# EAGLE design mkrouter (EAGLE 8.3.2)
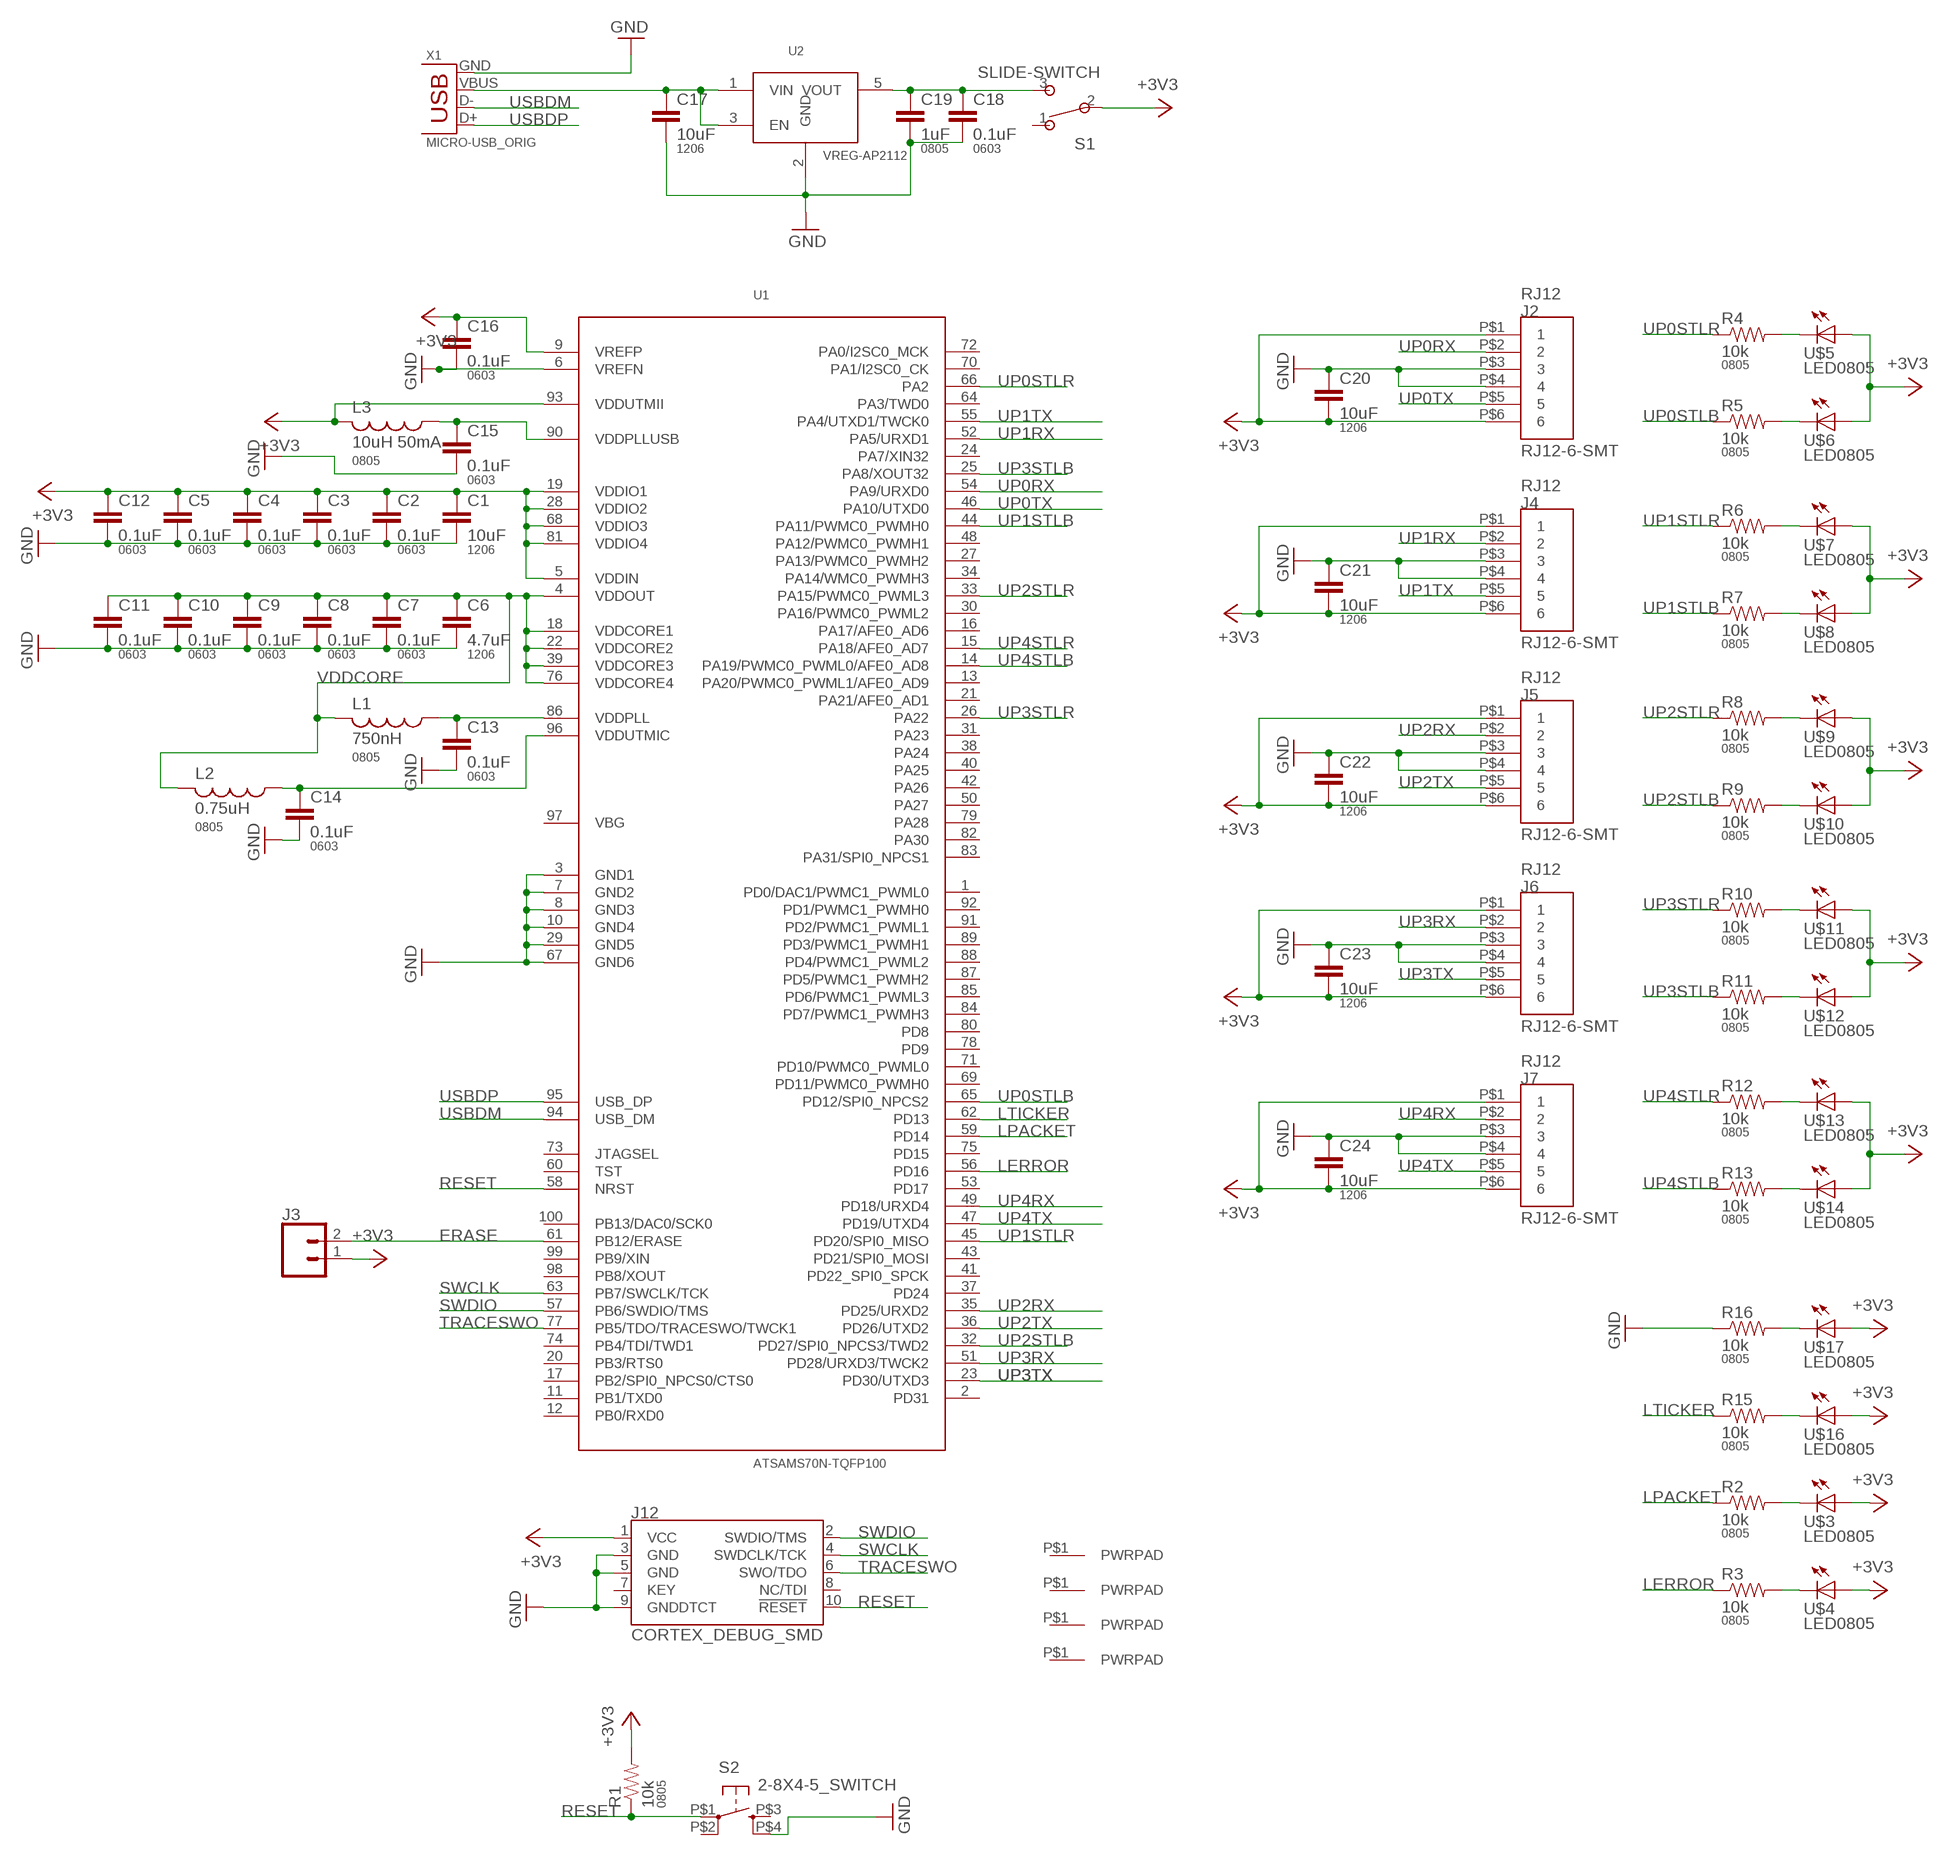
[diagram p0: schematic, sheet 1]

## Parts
C1  10uF  CAP1206  [1206]
C2  0.1uF  CAP0603-CAP  [0603-CAP]
C3  0.1uF  CAP0603-CAP  [0603-CAP]
C4  0.1uF  CAP0603-CAP  [0603-CAP]
C5  0.1uF  CAP0603-CAP  [0603-CAP]
C6  4.7uF  CAP1206  [1206]
C7  0.1uF  CAP0603-CAP  [0603-CAP]
C8  0.1uF  CAP0603-CAP  [0603-CAP]
C9  0.1uF  CAP0603-CAP  [0603-CAP]
C10  0.1uF  CAP0603-CAP  [0603-CAP]
C11  0.1uF  CAP0603-CAP  [0603-CAP]
C12  0.1uF  CAP0603-CAP  [0603-CAP]
C13  0.1uF  CAP0603-CAP  [0603-CAP]
C14  0.1uF  CAP0603-CAP  [0603-CAP]
C15  0.1uF  CAP0603-CAP  [0603-CAP]
C16  0.1uF  CAP0603-CAP  [0603-CAP]
C17  10uF  CAP1206  [1206]
C18  0.1uF  CAP0603-CAP  [0603-CAP]
C19  1uF  CAP0805  [0805]
C20  10uF  CAP1206  [1206]
C21  10uF  CAP1206  [1206]
C22  10uF  CAP1206  [1206]
C23  10uF  CAP1206  [1206]
C24  10uF  CAP1206  [1206]
J2  RJ12-6-SMT  [RJ12-6-SMT]
J3  CONN_021X02_NO_SILK  [1X02_NO_SILK]
J4  RJ12-6-SMT  [RJ12-6-SMT]
J5  RJ12-6-SMT  [RJ12-6-SMT]
J6  RJ12-6-SMT  [RJ12-6-SMT]
J7  RJ12-6-SMT  [RJ12-6-SMT]
J8  PWRPADM3  [PWRPAD_3-25MM]
J9  PWRPADM3  [PWRPAD_3-25MM]
J10  PWRPADM3  [PWRPAD_3-25MM]
J11  PWRPADM3  [PWRPAD_3-25MM]
J12  CORTEX_DEBUG_SMD  [SAMTECH_FTSH-105-01]
L1  750nH  INDUCTOR-0805  [0805]
L2  0.75uH  INDUCTOR-0805  [0805]
L3  10uH 50mA  INDUCTOR-0805  [0805]
R1  10k  RESISTOR0805-RES  [0805]
R2  10k  RESISTOR0805-RES  [0805]
R3  10k  RESISTOR0805-RES  [0805]
R4  10k  RESISTOR0805-RES  [0805]
R5  10k  RESISTOR0805-RES  [0805]
R6  10k  RESISTOR0805-RES  [0805]
R7  10k  RESISTOR0805-RES  [0805]
R8  10k  RESISTOR0805-RES  [0805]
R9  10k  RESISTOR0805-RES  [0805]
R10  10k  RESISTOR0805-RES  [0805]
R11  10k  RESISTOR0805-RES  [0805]
R12  10k  RESISTOR0805-RES  [0805]
R13  10k  RESISTOR0805-RES  [0805]
R15  10k  RESISTOR0805-RES  [0805]
R16  10k  RESISTOR0805-RES  [0805]
S1  SLIDE-SWITCH  [AYZ0102AGRLC]
S2  2-8X4-5_SWITCH  [TACT-SWITCH-KMR6]
U1  ATSAMS70N-TQFP100  [TQFP100-14X14]
U2  VREG-AP2112  [SOT23-5]
U$3  LED0805  [LED0805]
U$4  LED0805  [LED0805]
U$5  LED0805  [LED0805]
U$6  LED0805  [LED0805]
U$7  LED0805  [LED0805]
U$8  LED0805  [LED0805]
U$9  LED0805  [LED0805]
U$10  LED0805  [LED0805]
U$11  LED0805  [LED0805]
U$12  LED0805  [LED0805]
U$13  LED0805  [LED0805]
U$14  LED0805  [LED0805]
U$16  LED0805  [LED0805]
U$17  LED0805  [LED0805]
X1  MICRO-USB_ORIG  [DX4R005HJ5]

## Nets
+3V3: C1.1 C2.1 C3.1 C4.1 C5.1 C12.1 C16.1 C20.2 C21.2 C22.2 C23.2 C24.2 J2.P$1 J2.P$6 J3.1 J4.P$1 J4.P$6 J5.P$1 J5.P$6 J6.P$1 J6.P$6 J7.P$1 J7.P$6 J12.1(VCC) L3.2 R1.2 S1.2 U1.5(VDDIN) U1.9(VREFP) U1.19(VDDIO1) U1.28(VDDIO2) U1.68(VDDIO3) U1.81(VDDIO4) U1.93(VDDUTMII) U$3.1(A) U$4.1(A) U$5.1(A) U$6.1(A) U$7.1(A) U$8.1(A) U$9.1(A) U$10.1(A) U$11.1(A) U$12.1(A) U$13.1(A) U$14.1(A) U$16.1(A) U$17.1(A)
ERASE: J3.2 U1.61(PB12/ERASE)
GND: C1.2 C2.2 C3.2 C4.2 C5.2 C6.2 C7.2 C8.2 C9.2 C10.2 C11.2 C12.2 C13.2 C14.2 C15.2 C16.2 C17.2 C18.2 C19.2 C20.1 C21.1 C22.1 C23.1 C24.1 J2.P$3 J2.P$4 J4.P$3 J4.P$4 J5.P$3 J5.P$4 J6.P$3 J6.P$4 J7.P$3 J7.P$4 J12.3(GND) J12.5(GND) J12.9(GNDDTCT) R16.1 S2.P$4(S1) U1.3(GND1) U1.6(VREFN) U1.7(GND2) U1.8(GND3) U1.10(GND4) U1.29(GND5) U1.67(GND6) U2.2(GND) X1.GND
LERROR: R3.1 U1.56(PD16)
LPACKET: R2.1 U1.59(PD14)
LTICKER: R15.1 U1.62(PD13)
N$1: C13.1 L1.1 U1.86(VDDPLL)
N$2: R7.2 U$8.2(C)
N$3: C14.1 L2.1 U1.96(VDDUTMIC)
N$4: C17.1 U2.1(VIN) U2.3(EN) X1.VBUS
N$5: C15.1 L3.1 U1.90(VDDPLLUSB)
N$6: R5.2 U$6.2(C)
N$7: C18.1 C19.1 S1.3 U2.5(VOUT)
N$8: R4.2 U$5.2(C)
N$9: R6.2 U$7.2(C)
N$10: R9.2 U$10.2(C)
N$11: R8.2 U$9.2(C)
N$12: R11.2 U$12.2(C)
N$13: R10.2 U$11.2(C)
N$14: R13.2 U$14.2(C)
N$15: R12.2 U$13.2(C)
N$16: R2.2 U$3.2(C)
N$17: R3.2 U$4.2(C)
N$22: R15.2 U$16.2(C)
N$23: R16.2 U$17.2(C)
RESET: J12.10(!RESET) R1.1 S2.P$1(P) U1.58(NRST)
SWCLK: J12.4(SWDCLK/TCK) U1.63(PB7/SWCLK/TCK)
SWDIO: J12.2(SWDIO/TMS) U1.57(PB6/SWDIO/TMS)
TRACESWO: J12.6(SWO/TDO) U1.77(PB5/TDO/TRACESWO/TWCK1)
UP0RX: J2.P$2 U1.54(PA9/URXD0)
UP0STLB: R5.1 U1.65(PD12/SPI0_NPCS2)
UP0STLR: R4.1 U1.66(PA2)
UP0TX: J2.P$5 U1.46(PA10/UTXD0)
UP1RX: J4.P$2 U1.52(PA5/URXD1)
UP1STLB: R7.1 U1.44(PA11/PWMC0_PWMH0)
UP1STLR: R6.1 U1.45(PD20/SPI0_MISO)
UP1TX: J4.P$5 U1.55(PA4/UTXD1/TWCK0)
UP2RX: J5.P$2 U1.35(PD25/URXD2)
UP2STLB: R9.1 U1.32(PD27/SPI0_NPCS3/TWD2)
UP2STLR: R8.1 U1.33(PA15/PWMC0_PWML3)
UP2TX: J5.P$5 U1.36(PD26/UTXD2)
UP3RX: J6.P$2 U1.51(PD28/URXD3/TWCK2)
UP3STLB: R11.1 U1.25(PA8/XOUT32)
UP3STLR: R10.1 U1.26(PA22)
UP3TX: J6.P$5 U1.23(PD30/UTXD3)
UP4RX: J7.P$2 U1.49(PD18/URXD4)
UP4STLB: R13.1 U1.14(PA19/PWMC0_PWML0/AFE0_AD8)
UP4STLR: R12.1 U1.15(PA18/AFE0_AD7)
UP4TX: J7.P$5 U1.47(PD19/UTXD4)
USBDM: U1.94(USB_DM) X1.D-
USBDP: U1.95(USB_DP) X1.D+
VDDCORE: C6.1 C7.1 C8.1 C9.1 C10.1 C11.1 L1.2 L2.2 U1.4(VDDOUT) U1.18(VDDCORE1) U1.22(VDDCORE2) U1.39(VDDCORE3) U1.76(VDDCORE4)
Unconnected: J8.P$1(PWRPAD) J9.P$1(PWRPAD) J10.P$1(PWRPAD) J11.P$1(PWRPAD) J12.7(KEY) J12.8(NC/TDI) S1.1 S2.P$2(P1) S2.P$3(S) U1.1(PD0/DAC1/PWMC1_PWML0) U1.2(PD31) U1.11(PB1/TXD0) U1.12(PB0/RXD0) U1.13(PA20/PWMC0_PWML1/AFE0_AD9) U1.16(PA17/AFE0_AD6) U1.17(PB2/SPI0_NPCS0/CTS0) U1.20(PB3/RTS0) U1.21(PA21/AFE0_AD1) U1.24(PA7/XIN32) U1.27(PA13/PWMC0_PWMH2) U1.30(PA16/PWMC0_PWML2) U1.31(PA23) U1.34(PA14/WMC0_PWMH3) U1.37(PD24) U1.38(PA24) U1.40(PA25) U1.41(PD22_SPI0_SPCK) U1.42(PA26) U1.43(PD21/SPI0_MOSI) U1.48(PA12/PWMC0_PWMH1) U1.50(PA27) U1.53(PD17) U1.60(TST) U1.64(PA3/TWD0) U1.69(PD11/PWMC0_PWMH0) U1.70(PA1/I2SC0_CK) U1.71(PD10/PWMC0_PWML0) U1.72(PA0/I2SC0_MCK) U1.73(JTAGSEL) U1.74(PB4/TDI/TWD1) U1.75(PD15) U1.78(PD9) U1.79(PA28) U1.80(PD8) U1.82(PA30) U1.83(PA31/SPI0_NPCS1) U1.84(PD7/PWMC1_PWMH3) U1.85(PD6/PWMC1_PWML3) U1.87(PD5/PWMC1_PWMH2) U1.88(PD4/PWMC1_PWML2) U1.89(PD3/PWMC1_PWMH1) U1.91(PD2/PWMC1_PWML1) U1.92(PD1/PWMC1_PWMH0) U1.97(VBG) U1.98(PB8/XOUT) U1.99(PB9/XIN) U1.100(PB13/DAC0/SCK0)

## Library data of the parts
C1 C6 C17 C20-C24 = borkedlabs-passives:CAP: Capacitor; PACKAGE: 1206
C2-C5 C7-C16 C18 = borkedlabs-passives:CAP: Capacitor; PACKAGE: 0603
C19 = borkedlabs-passives:CAP: Capacitor; PACKAGE: 0805
J2 J4-J7 = connector:RJ12-6-SMT
J3 = SparkFun-Connectors:CONN_02: Multi connection point. Often used as Generic Header-pin footprint for 0.1 inch spaced/style header connections
J8-J11 = power:PWRPAD
J12 = SparkFun-Connectors:CORTEX_DEBUG: Cortex Debug Connector - 10 pin Supports JTAG debug, Serial Wire debug, and Serial Wire Viewer. PTH and SMD connector options available. General Connector Information Products: PTH Connector -via Digi-Key SparkFun PSoc SparkFun T
L1-L3 = borkedlabs-passives:INDUCTOR; PACKAGE: 0805
R1-R13 R15 R16 = borkedlabs-passives:RESISTOR: Resistor; PACKAGE: 0805
S1 = fab:SLIDE-SWITCH: SMD slide-switch AYZ0102AGRLC as found in the fablab inventory. Includes the mounting holes. Made by Zaerc.
S2 = fab:2-8X4-5_SWITCH
U1 = atsam:ATSAMS70N-TQFP100
U2 = power:VREG-AP2112
U$3-U$14 U$16 U$17 = lights:LED: LED
X1 = fab:MICRO-USB: SMD micro USB connector as found in the fablab inventory. Three footprint variants included: original, as described by manufacturer's datasheet for milling with the 1/100" bit for milling with the 1/64" bit Made by Zaerc.

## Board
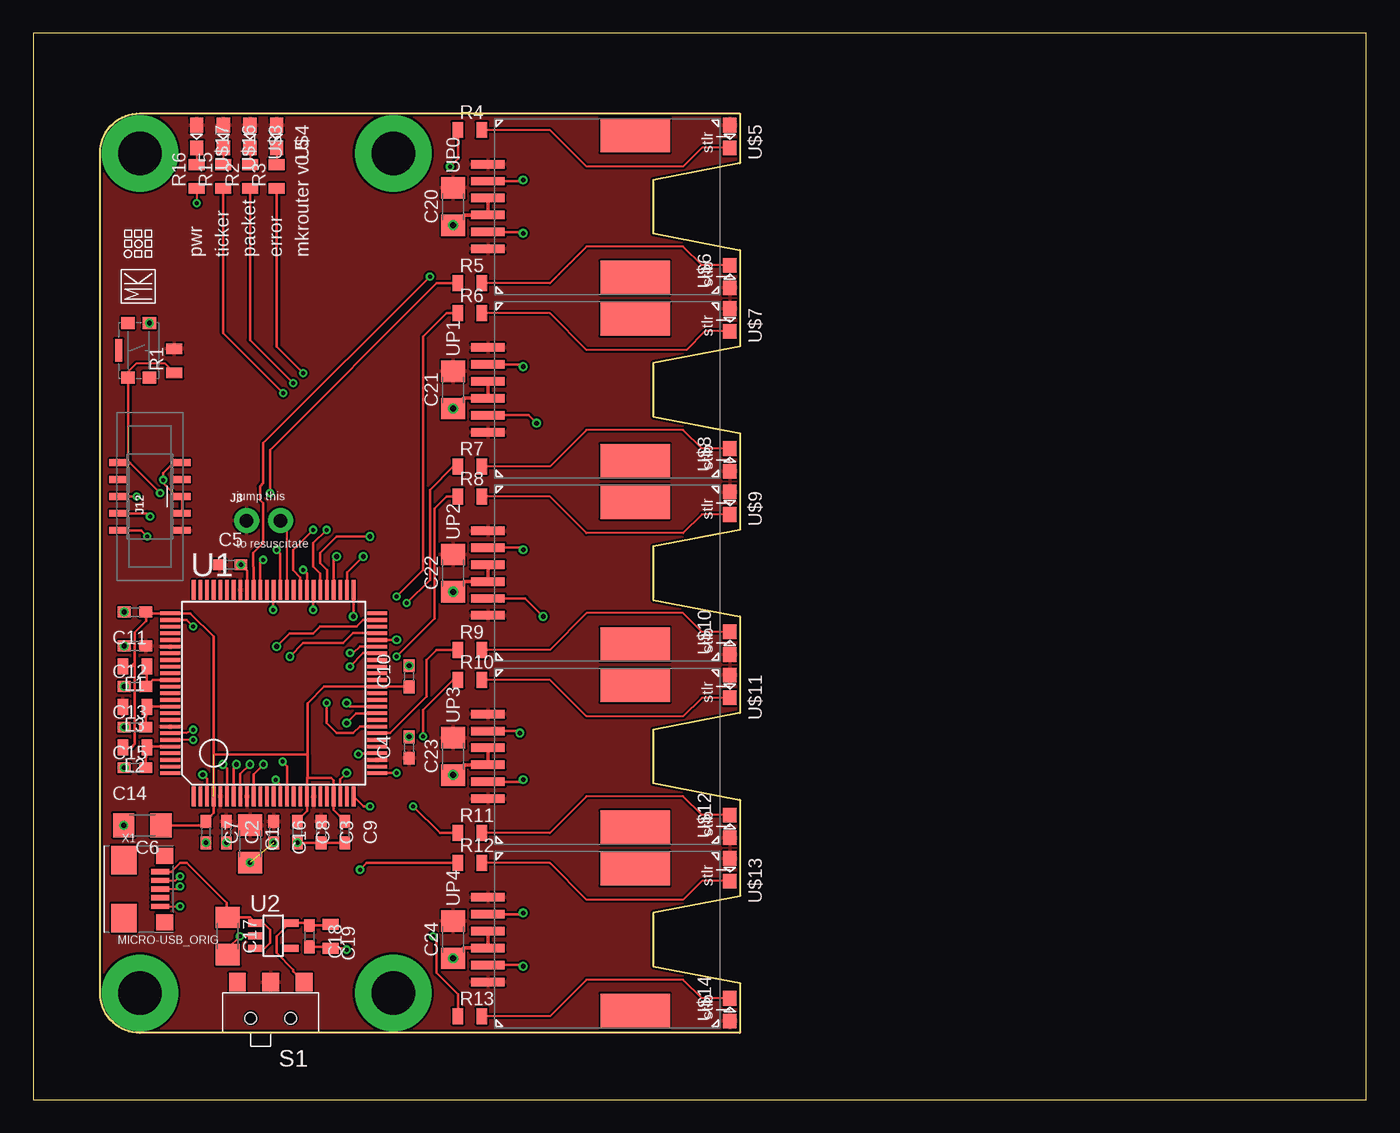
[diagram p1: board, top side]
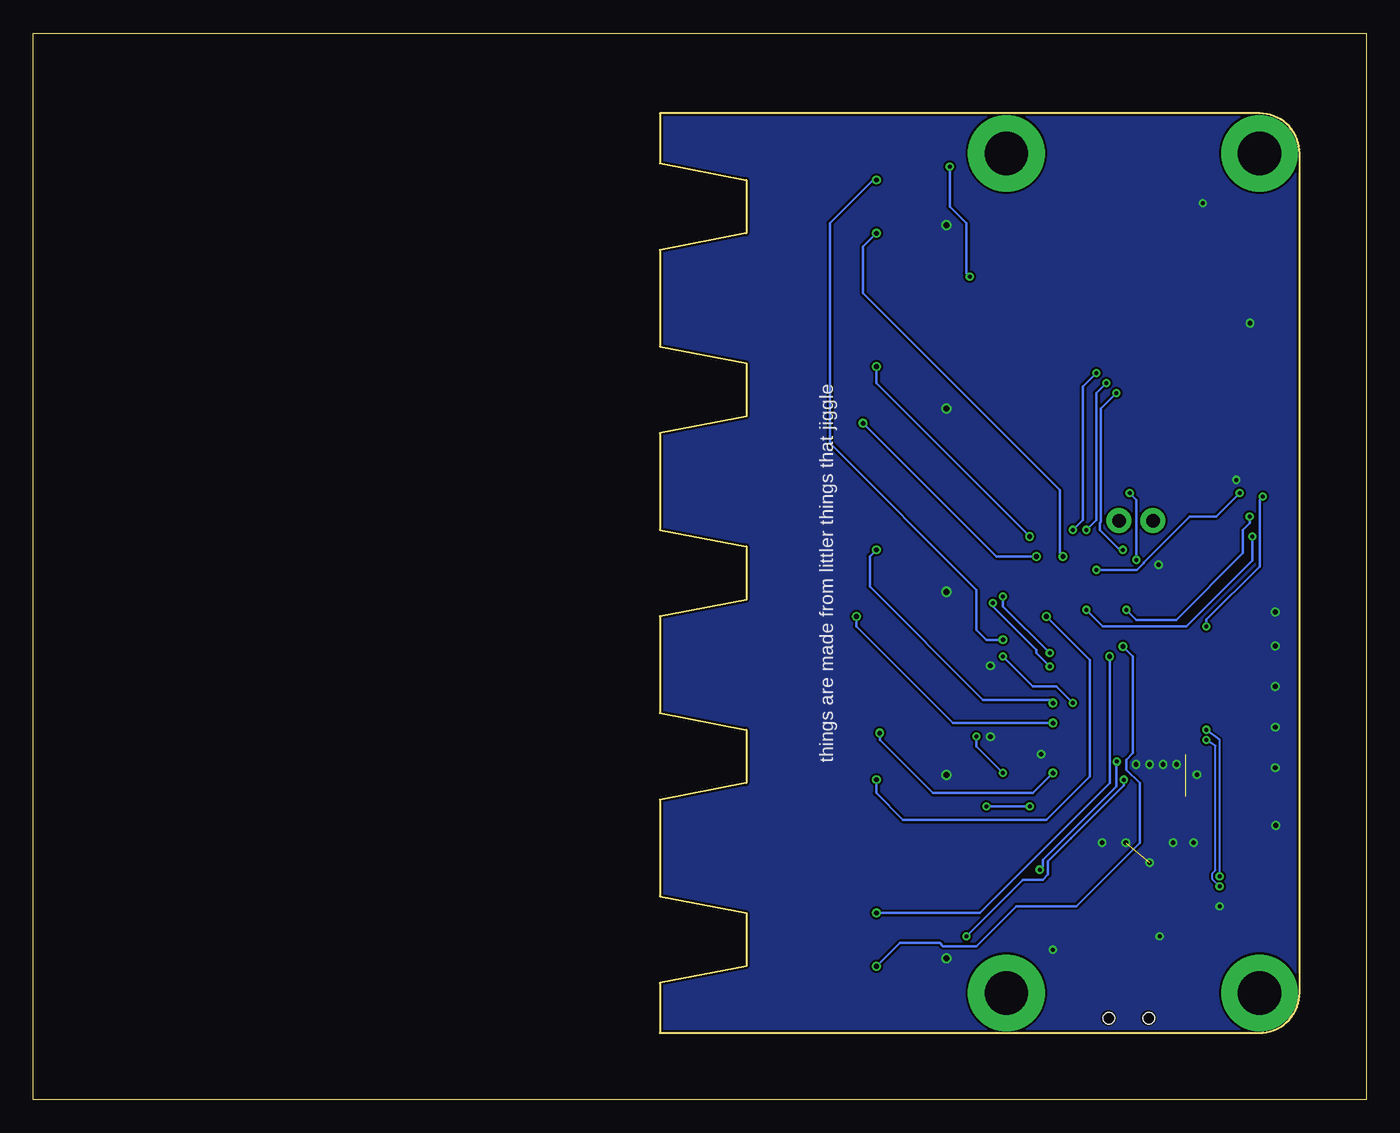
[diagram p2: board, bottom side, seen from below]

Size 100 x 80 mm. Coordinates in mm from the lower left corner, seen from the top.
Outline: 0,0 100,0 100,80 0,80 0,0
Outline: 8,74 53,74 53,70.25 46.5,69 46.5,65 53,63.75 53,56.5 46.5,55.25 46.5,51.25 53,50 53,42.75 46.5,41.5 46.5,37.5 53,36.25 53,29 46.5,27.75 46.5,23.75 53,22.5 53,15.25 46.5,14 46.5,10 53,8.75 53,5 8,5 arc-90 5,8 5,71 arc-90 8,74
Copper layers (1*16): Top 0.035mm / dielectric 1.5mm / Bottom 0.035mm
Design rules "default *": minimum track width 6mil, minimum drill 0.3mm, track to track 6mil, track to pad 6mil, pad to pad 6mil, via to via 6mil, smd to smd 6mil, copper to edge 6mil, drill to drill 6mil, minimum pad ring 10mil, minimum via ring 6mil, stop-mask expansion 4mil, vias tented up to drill 20mil, thermal gap 6mil

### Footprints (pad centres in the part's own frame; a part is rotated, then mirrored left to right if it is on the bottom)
1206 = smd 1.6 x 1.8: 1 -1.4,0; 2 1.4,0
0603-CAP = smd 0.96 x 0.8: 1 -0.8,0; 2 0.8,0
0805 = smd 0.8 x 1.2: 1 -0.9,0; 2 0.9,0
RJ12-6-SMT = smd 0.635 x 2.54: P$1 -3.175,17.399; P$2 -1.905,17.399; P$3 -0.635,17.399; P$4 0.635,17.399; P$5 1.905,17.399; P$6 3.175,17.399 | smd 2.54 x 5.207: P$7 -5.334,6.35; P$8 5.334,6.35
1X02_NO_SILK = drill 1.016 pad 1.88: 1 0,0; 2 2.54,0
PWRPAD_3-25MM = drill 3.25 pad 5.75: P$1 0,0
SAMTECH_FTSH-105-01 = smd 0.508 x 1.27: 1 -2.54,-2.413; 2 -2.54,2.413; 3 -1.27,-2.413; 4 -1.27,2.413; 5 0,-2.413; 6 0,2.413; 7 1.27,-2.413; 8 1.27,2.413; 9 2.54,-2.413; 10 2.54,2.413
AYZ0102AGRLC = smd 1.27 x 1.397: 1 2.5,-2.3; 2 0,-2.3; 3 -2.5,-2.3 | hole 0.85: -1.5,0.4; 1.5,0.4
TACT-SWITCH-KMR6 = smd 0.9 x 1: P$1 -2.05,0.8; P$2 2.05,0.8; P$3 -2.05,-0.8; P$4 2.05,-0.8 | smd 1.7 x 0.55: P$5 0,1.5
TQFP100-14X14 = smd 0.27 x 1.5: 1 -6,-7.75; 2 -5.5,-7.75; 3 -5,-7.75; 4 -4.5,-7.75; 5 -4,-7.75; 6 -3.5,-7.75; 7 -3,-7.75; 8 -2.5,-7.75; 9 -2,-7.75; 10 -1.5,-7.75; 11 -1,-7.75; 12 -0.5,-7.75; 13 0,-7.75; 14 0.5,-7.75; 15 1,-7.75; 16 1.5,-7.75; 17 2,-7.75; 18 2.5,-7.75; 19 3,-7.75; 20 3.5,-7.75; 21 4,-7.75; 22 4.5,-7.75; 23 5,-7.75; 24 5.5,-7.75; 25 6,-7.75; 51 6,7.75; 52 5.5,7.75; 53 5,7.75; 54 4.5,7.75; 55 4,7.75; 56 3.5,7.75; 57 3,7.75; 58 2.5,7.75; 59 2,7.75; 60 1.5,7.75; 61 1,7.75; 62 0.5,7.75; 63 0,7.75; 64 -0.5,7.75; 65 -1,7.75; 66 -1.5,7.75; 67 -2,7.75; 68 -2.5,7.75; 69 -3,7.75; 70 -3.5,7.75; 71 -4,7.75; 72 -4.5,7.75; 73 -5,7.75; 74 -5.5,7.75; 75 -6,7.75 | smd 1.5 x 0.27: 26 7.75,-6; 27 7.75,-5.5; 28 7.75,-5; 29 7.75,-4.5; 30 7.75,-4; 31 7.75,-3.5; 32 7.75,-3; 33 7.75,-2.5; 34 7.75,-2; 35 7.75,-1.5; 36 7.75,-1; 37 7.75,-0.5; 38 7.75,0; 39 7.75,0.5; 40 7.75,1; 41 7.75,1.5; 42 7.75,2; 43 7.75,2.5; 44 7.75,3; 45 7.75,3.5; 46 7.75,4; 47 7.75,4.5; 48 7.75,5; 49 7.75,5.5; 50 7.75,6; 76 -7.75,6; 77 -7.75,5.5; 78 -7.75,5; 79 -7.75,4.5; 80 -7.75,4; 81 -7.75,3.5; 82 -7.75,3; 83 -7.75,2.5; 84 -7.75,2; 85 -7.75,1.5; 86 -7.75,1; 87 -7.75,0.5; 88 -7.75,0; 89 -7.75,-0.5; 90 -7.75,-1; 91 -7.75,-1.5; 92 -7.75,-2; 93 -7.75,-2.5; 94 -7.75,-3; 95 -7.75,-3.5; 96 -7.75,-4; 97 -7.75,-4.5; 98 -7.75,-5; 99 -7.75,-5.5; 100 -7.75,-6
SOT23-5 = smd 0.533 x 1.194: 1 -0.95,-1.306; 2 0,-1.306; 3 0.95,-1.306; 4 0.95,1.306; 5 -0.95,1.306
LED0805 = smd 1.1 x 1: 1 -0.85,0; 2 0.85,0
DX4R005HJ5 = smd 0.4 x 1.35: D+ 0,1.6; D- -0.65,1.6; GND 1.3,1.6; ID 0.65,1.6; VBUS -1.3,1.6 | smd 1.2 x 1.3: GND@1 -2.5,1.95; GND@2 2.5,1.95 | smd 2.15 x 1.9: GND@3 -2.175,-1.1; GND@4 2.175,-1.1

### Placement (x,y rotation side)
C1  16.26,19.18 270 top
C2  14.48,20.07 270 top
C3  21.59,20.07 270 top
C4  28.19,26.42 90 top
C5  14.77,40.12 0 top
C6  8.18,20.57 180 top
C7  12.95,20.07 270 top
C8  19.81,20.07 270 top
C9  23.37,20.07 270 top
C10  28.19,31.75 90 top
C11  7.62,36.58 180 top
C12  7.62,34.04 180 top
C13  7.62,30.99 180 top
C14  7.62,24.89 180 top
C15  7.62,27.94 180 top
C16  18.03,20.07 270 top
C17  14.58,12.26 270 top
C18  20.72,12.26 270 top
C19  22.29,12.25 270 top
C20  31.5,67 90 top
C21  31.5,53.25 90 top
C22  31.5,39.5 90 top
C23  31.5,25.75 90 top
C24  31.5,12 90 top
J2  51.5,67 90 top
J3  16,43.43 0 top
J4  51.5,53.25 90 top
J5  51.5,39.5 90 top
J6  51.5,25.75 90 top
J7  51.5,12 90 top
J8  8,8 0 top
J9  27,8 0 top
J10  27,71 0 top
J11  8,71 0 top
J12  8.75,45.25 90 top
L1  7.62,32.51 180 top
L2  7.62,26.42 180 top
L3  7.62,29.46 180 top
R1  10.58,55.43 90 top
R2  16.25,69.25 90 top
R3  18.25,69.25 90 top
R4  32.75,72.75 0 top
R5  32.75,61.25 0 top
R6  32.75,59 0 top
R7  32.75,47.5 0 top
R8  32.75,45.25 0 top
R9  32.75,33.75 0 top
R10  32.75,31.5 0 top
R11  32.75,20 0 top
R12  32.75,17.75 0 top
R13  32.75,6.25 0 top
R15  14.25,69.25 90 top
R16  12.25,69.25 90 top
S1  17.81,6.5 180 top
S2  7.9,56.21 90 top
U1  18.03,30.48 0 top
U2  18.01,12.29 270 top
U$1  [CBA-SILK-LOGO]  7.87,64.22 90 top
U$2  [MK-LOGO-SILK]  7.87,61.01 90 top
U$3  16.25,72.25 270 top
U$4  18.25,72.25 270 top
U$5  52.25,72.25 270 top
U$6  52.25,61.75 90 top
U$7  52.25,58.5 270 top
U$8  52.25,48 90 top
U$9  52.25,44.75 270 top
U$10  52.25,34.25 90 top
U$11  52.25,31 270 top
U$12  52.25,20.5 90 top
U$13  52.25,17.25 270 top
U$14  52.25,6.75 90 top
U$16  14.25,72.25 270 top
U$17  12.25,72.25 270 top
X1  7.9,15.8 270 top

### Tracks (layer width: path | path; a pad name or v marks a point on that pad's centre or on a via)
+3V3
  pour Top (rank 2): 5,74 5,5 53,5 53,74
ERASE
  Top 0.152: U1.61 19.03,42.94 J3.2
GND  (via drill 0.3, 0.35, 0.45)  (1 unrouted)
  Top 0.152: X1.GND v11,14.5 | R16.1 v12.25,67.25
  Top 0.2: U2.2 15.54,12.29 v15.5,12.25
  Top 0.203: U1.3 13.03,24.05 v12.7,24.38 | U1.6 14.53,24.84 v14.22,25.15 | U1.7 15.03,24.94 v15.24,25.15 | U1.8 15.53,24.42 v16.26,25.15 | U1.10 16.53,24.41 v17.27,25.15 | U1.29 24.46,25.98 v24.38,25.91 | C9.2 C3.2 C8.2 | C17.2 14.58,11.33 v15.5,12.25 | C18.2 22.18,11.46 C19.2 23.4,11.35 v23.5,11.25 | J12.3 J12.5 10.75,45.25 9.75,46.25 v9.75,46.5 9.75,47 10.54,47.79 J12.9 | U1.67 16.03,39.66 C5.2
  Top 0.254: J2.P$4 J2.P$3 32.27,66.36 C20.1 | J4.P$4 J4.P$3 32.27,52.62 C21.1 | J5.P$4 J5.P$3 32.27,38.87 C22.1 | J6.P$4 J6.P$3 32.27,25.11 C23.1 | J7.P$4 J7.P$3 32.27,11.37 C24.1
  other vias: 6.82,36.58 6.82,34.04 6.82,30.99 6.82,27.94 6.82,24.89 15.57,40.12 6.78,20.57 12.95,19.27 14.48,19.27 16.26,17.78 18.03,19.27 19.81,19.27 28.19,27.22 28.19,32.55 8.7,58.26 31.5,65.6 31.5,51.85 31.5,38.1 31.5,24.35 31.5,10.6
  pour Bottom: 5,74 53,74 53,5 5,5
LERROR  (via drill 0.3)
  Top 0.203: R3.1 18.25,56.5 v20.25,54.5 | v22,42.75 21,41.75 21,40 21.53,39.47 U1.56
  Bottom 0.203: v20.25,54.5 21.25,53.5 21.25,43.5 v22,42.75
LPACKET  (via drill 0.3)
  Top 0.203: R2.1 16.25,57 v19.5,53.75 | v21,42.75 19.5,41.25 19.5,39.71 20.03,39.18 U1.59
  Bottom 0.203: v19.5,53.75 20.25,53 20.25,43.5 v21,42.75
LTICKER  (via drill 0.3)
  Top 0.203: U1.62 18.53,40.97 v18.25,41.25 | v18.75,53 14.25,57.5 R15.1
  Bottom 0.203: v18.25,41.25 18.5,41.25 20,42.75 20,43.25 19.89,43.35 19.89,51.86 v18.75,53
N$1
  Top 0.203: 8.52,31.04 L1.1 | 8.52,31.04 C13.1 | U1.86 8.96,31.48 8.52,31.04
N$2
  Top 0.152: U$8.2 50.15,48.85 48.75,50.25 41.5,50.25 38.75,47.5 R7.2
N$3
  Top 0.203: U1.96 8.58,26.48 L2.1 8.47,26.37 C14.1
N$4
  Top 0.2: X1.VBUS 10.35,17.1 11,17.75 11.5,17.75 14.5,14.75 14.5,13.75 C17.1 16.28,13.66 U2.1 17.26,13.24 17.75,12.75 17.75,11.75 17.25,11.25 16.79,11.25 U2.3
N$5
  Top 0.203: U1.90 8.54,29.48 L3.1 8.47,29.41 C15.1
N$6
  Top 0.152: U$6.2 50.15,62.6 48.75,64 41.5,64 38.75,61.25 R5.2
N$7
  Top 0.2: C19.1 22.2,13.06 C18.1 20.54,13.24 U2.5 19.24,13.24 18.25,12.25 18.25,11 19.5,9.75 19.5,9.61 S1.3
N$8
  Top 0.152: U$5.2 50.15,71.4 48.75,70 41.5,70 38.75,72.75 R4.2
N$9
  Top 0.152: U$7.2 50.4,57.65 49,56.25 41.5,56.25 38.75,59 R6.2
N$10
  Top 0.152: U$10.2 50.15,35.1 48.75,36.5 41.5,36.5 38.75,33.75 R9.2
N$11
  Top 0.152: U$9.2 50.15,43.9 48.75,42.5 41.5,42.5 38.75,45.25 R8.2
N$12
  Top 0.152: U$12.2 50.15,21.35 48.75,22.75 41.5,22.75 38.75,20 R11.2
N$13
  Top 0.152: U$11.2 50.15,30.15 48.75,28.75 41.5,28.75 38.75,31.5 R10.2
N$14
  Top 0.152: U$14.2 50.15,7.6 48.75,9 41.5,9 38.75,6.25 R13.2
N$15
  Top 0.152: U$13.2 50.15,16.4 48.75,15 41.5,15 38.75,17.75 R12.2
N$16
  Top 0.152: U$3.2 R2.2
N$17
  Top 0.152: U$4.2 R3.2
N$22
  Top 0.152: U$16.2 R15.2
N$23
  Top 0.152: U$17.2 R16.2
RESET  (via drill 0.3)
  Top 0.152: S2.P$1 7.1,54.6 7.75,55.25 9.86,55.25 R1.1
  Top 0.203: U1.58 20.53,39.47 v20.25,39.75 | 7.25,47.75 v9.5,45.5 | 7.25,47.75 6.38,47.75 J12.10 | S2.P$1 7.1,47.9 7.25,47.75
  Bottom 0.203: v20.25,39.75 17.21,39.75 16.69,40.27 16.69,40.31 13.25,43.75 11.25,43.75 v9.5,45.5
SWCLK  (via drill 0.3)
  Top 0.203: J12.4 8.52,43.98 v8.75,43.75 | v18,36.75 18,38.2 U1.63
  Bottom 0.203: v8.75,43.75 8.75,43.25 9.25,42.75 9.25,41 14.25,36 17.25,36 v18,36.75
SWDIO  (via drill 0.3)
  Top 0.203: J12.2 8.1,42.71 v8.56,42.25 | v21,36.75 21,38.2 U1.57
  Bottom 0.203: v8.56,42.25 8.56,40.44 13.5,35.5 19.75,35.5 v21,36.75
TRACESWO  (via drill 0.3)
  Top 0.203: U1.77 11.49,35.98 v11.99,35.49 | v7.75,45.25 J12.6
  Bottom 0.203: v11.99,35.49 11.99,36.01 8,40 8,45 v7.75,45.25
UP0RX  (via drill 0.35)
  Top 0.203: J2.P$2 36.66,65.09 v36.75,65 | U1.54 22.53,40.53 v22.75,40.75
  Bottom 0.203: v36.75,65 37.75,64 37.75,60.5 23,45.75 23,41 v22.75,40.75
UP0STLB  (via drill 0.3)
  Top 0.203: U1.65 17.03,40.28 v17.25,40.5 | v17.75,45.5 17.75,48.75 30.25,61.25 R5.1
  Bottom 0.203: v17.25,40.5 17.25,45 v17.75,45.5
UP0STLR  (via drill 0.3)
  Top 0.203: R4.1 31.85,70.6 v31.25,70 | v29.75,61.75 17.25,49.25 17.25,46.25 17,46 17,45 17.25,44.75 17.25,41.75 16.5,41 16.5,40 16.53,39.97 U1.66
  Bottom 0.203: v31.25,70 31.25,67 30,65.75 30,62 v29.75,61.75
UP0TX  (via drill 0.35)
  Top 0.203: J2.P$5 36.66,68.91 v36.75,69 | v27.25,34.5 25.8,34.5 U1.46
  Bottom 0.203: v36.75,69 37,69 40.25,65.75 40.25,49.25 29.25,38.25 29.25,35.25 28.5,34.5 v27.25,34.5
UP1RX  (via drill 0.35)
  Top 0.203: J4.P$2 37.16,51.34 v37.75,50.75 | U1.52 23.53,39.53 v24.75,40.75
  Bottom 0.203: v37.75,50.75 27.75,40.75 v24.75,40.75
UP1STLB  (via drill 0.3)
  Top 0.203: R7.1 31.5,47.5 29.75,45.75 29.75,39 v28,37.25 | v23.75,32.5 24.75,33.5 25.76,33.5 U1.44
  Bottom 0.203: v28,37.25 28,37 24.75,33.75 24.75,33.5 v23.75,32.5
UP1STLR  (via drill 0.3)
  Top 0.203: R6.1 31,59 29.25,57.25 29.25,39.75 v27.25,37.75 | v23.75,33.5 24,33.5 24.5,34 25.76,34 U1.45
  Bottom 0.203: v27.25,37.75 27.25,37 v23.75,33.5
UP1TX  (via drill 0.35)
  Top 0.203: J4.P$5 36.59,55.16 v36.75,55 | v25.25,42.25 22.75,42.25 21.5,41 21.5,40.25 22.03,39.72 U1.55
  Bottom 0.203: v36.75,55 36.75,53.75 v25.25,42.25
UP2RX  (via drill 0.35)
  Top 0.203: J5.P$2 36.91,37.59 v38.25,36.25 | U1.35 24.23,28.98 v23.5,28.25
  Bottom 0.203: v38.25,36.25 38.25,35.5 31,28.25 v23.5,28.25
UP2STLB
  Top 0.203: R9.1 30.25,33.75 29.5,33 29.5,30.25 26.75,27.5 25.8,27.5 U1.32
UP2STLR  (via drill 0.3)
  Top 0.203: R8.1 31,45.25 30.11,44.36 30.11,36.11 v27.25,33.25 | v22,29.75 22,28.25 22.75,27.5 24,27.5 24.5,28 25.76,28 U1.33
  Bottom 0.203: v27.25,33.25 25,31 23.25,31 v22,29.75
UP2TX  (via drill 0.35)
  Top 0.203: J5.P$5 36.59,41.41 v36.75,41.25 | U1.36 23.77,29.48 v23.5,29.75
  Bottom 0.203: v36.75,41.25 37.25,40.75 37.25,38.5 28.75,30 23.75,30 v23.5,29.75
UP3RX  (via drill 0.35)
  Top 0.203: J6.P$2 36.59,23.84 v36.75,24 | U1.51 24.03,36.28 v24,36.25
  Bottom 0.203: v36.75,24 36.75,23 34.75,21 24,21 20.75,24.25 20.75,33 v24,36.25
UP3STLB  (via drill 0.3)
  Top 0.203: R11.1 30.5,20 v28.5,22 | v25.25,22 24.76,22 U1.25
  Bottom 0.203: v28.5,22 v25.25,22
UP3STLR  (via drill 0.3)
  Top 0.203: R10.1 31.5,31.5 29.25,29.25 v29.25,27.25 | v27.25,24.5 25.8,24.5 U1.26
  Bottom 0.203: v29.25,27.25 29.25,26.5 v27.25,24.5
UP3TX  (via drill 0.35)
  Top 0.203: J6.P$5 36.34,27.66 v36.5,27.5 | U1.23 23.03,24.03 v23.5,24.5
  Bottom 0.203: v36.5,27.5 36.5,27 32.5,23 25,23 v23.5,24.5
UP4RX  (via drill 0.35)
  Top 0.203: J7.P$2 36.66,10.1 v36.75,10 | U1.49 24.73,35.98 24.25,35.5 21.5,35.5 20.98,34.98 19.23,34.98 v18.25,34
  Bottom 0.203: v18.25,34 17.5,33.25 17.5,26 18,25.5 18,24.75 17,23.75 17,19.25 21.75,14.5 26.25,14.5 29.25,11.5 31.75,11.5 32,11.75 35,11.75 v36.75,10
UP4STLB  (via drill 0.3)
  Top 0.203: U1.14 18.53,23.66 v18.19,24 | R13.1 31.85,7.9 30.25,9.5 30.25,12 v30,12.25
  Bottom 0.203: v18.19,24 18.19,23.55 22.14,19.6 23.87,17.87 23.87,16.88 24.25,16.5 25.75,16.5 v30,12.25
UP4STLR  (via drill 0.3)
  Top 0.203: R12.1 25,17.75 v24.5,17.25 | U1.15 19.03,25.01 v18.69,25.35
  Bottom 0.203: v18.69,25.35 18.75,25.3 18.75,23.5 24.25,18 24.25,17.5 v24.5,17.25
UP4TX  (via drill 0.35)
  Top 0.203: J7.P$5 36.66,13.9 v36.75,14 | U1.47 25.76,35 24,35 23.25,34.25 20.25,34.25 v19.25,33.25
  Bottom 0.203: v36.75,14 29,14 19.25,23.75 v19.25,33.25
USBDM  (via drill 0.3)
  Top 0.152: X1.D- 10.7,16.45 v11,16.75 | v12,27.75 11.5,27.5 10.3,27.5 U1.94
  Bottom 0.152: v11,16.75 11,27 v12,27.75
USBDP  (via drill 0.3)
  Top 0.152: X1.D+ 10.8,15.8 v11,15.99 | v12,26.99 10.3,26.99 U1.95
  Bottom 0.152: v11,15.99 v11,16 11.53,16.53 11.53,16.97 11.3,17.2 11.3,26.55 v12,26.99
VDDCORE  (1 unrouted)
  Top 0.203: 7.62,32.77 7.62,35.05 8.47,35.9 C11.1 8.57,36.48 U1.76 11.78,36.48 13.53,34.73 U1.4 13.53,21.5 C7.1 12.62,20.58 C6.1 | 7.62,32.77 7.37,32.51 L1.2 | 7.62,32.77 7.62,26.67 7.37,26.42 L2.2 | C8.1 20.53,21.64 U1.18 20.53,24.13 | C9.1 22.53,21.75 U1.22 22.53,23.95 22.35,24.13 20.53,24.13 | 20.53,24.13 20.53,24.17 | 20.57,25.91 20.57,29.72 21.84,30.98 U1.39 28.11,30.98 C10.1 | 20.57,25.91 20.57,24.17 20.53,24.13 | 13.53,25.91 20.57,25.91

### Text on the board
tPlace: UP0 | pwr | ticker | packet | error | mkrouter v0.5 | UP1 | jump this | UP2 | to resuscitate | UP3 | UP4
bPlace: things are made from littler things that jiggle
